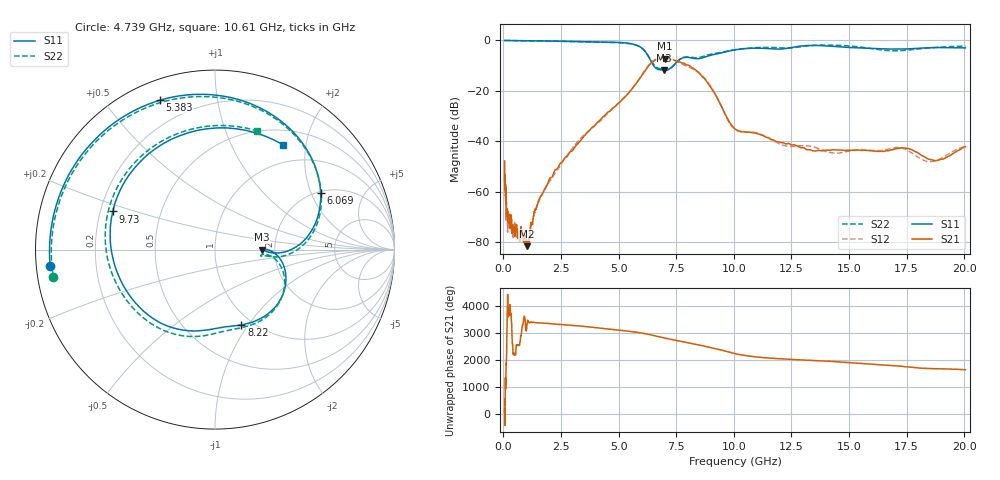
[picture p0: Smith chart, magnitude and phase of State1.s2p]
# Hz S DB R 50
!freq MagS11 AngS11 MagS21 AngS21 MagS12 AngS12 MagS22 AngS22
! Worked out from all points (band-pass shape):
!   1601 points, 50 MHz to 20.05 GHz, reference 50 ohm
!   highest |S21| = -7.19 dB at 7.024 GHz (marker M1); lowest = -81.5 dB at 1.016 GHz (marker M2)
!   |S21| within 3 dB of the highest: 6.292 GHz to 8.101 GHz (1.808 GHz wide, 25.1 % of centre)
!   lowest |S11| = -11.7 dB at 6.971 GHz (marker M3), VSWR 1.70, Z = 85.2 + j0.0103 ohm
!   |S11| at or under -10 dB: 6.519 GHz to 7.366 GHz (846.4 MHz wide, 12.2 % of centre)
!   |S22| runs from -11.8 to 0.0 dB; largest |S21 - S12| = 0.028
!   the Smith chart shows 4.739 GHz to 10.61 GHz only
!   S11 on the Smith chart (normalised r, x): 4.739 GHz: 0.04, -0.05; 5.383 GHz: 0.09, +0.69; 6.069 GHz: 2.06, +2.35; 8.22 GHz: 0.89, -0.93; 9.73 GHz: 0.25, +0.17; 10.61 GHz: 0.71, +1.61
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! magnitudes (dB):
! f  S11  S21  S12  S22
! 50 MHz  0.0  -47.8  -57.9  0.0
! 52.89 MHz  0.0  -55.3  -55.0  0.0
! 109 MHz  0.0  -61.2  -69.4  0.0
! 135.9 MHz  0.0  -68.4  -67.3  0.0
! 165.2 MHz  0.0  -68.3  -68.3  0.0
! 181.4 MHz  0.0  -68.6  -74.8  0.0
! 193.3 MHz  0.0  -69.3  -70.1  0.0
! 369.6 MHz  0.0  -75.1  -74.2  0.0
! 1.005 GHz  -0.1  -80.3  -79.9  -0.1
! 1.016 GHz  -0.1  -81.5  -81.0  -0.1
! 2.722 GHz  -0.3  -46.2  -46.1  -0.4
! 4.739 GHz  -0.7  -26.8  -27.0  -0.8
! 5.383 GHz  -1.0  -21.3  -21.3  -1.2
! 6.069 GHz  -3.5  -13.0  -12.8  -3.6
! 6.971 GHz  -11.7  -7.2  -7.0  -11.7
! 7.024 GHz  -11.7  -7.2  -7.0  -11.8
! 7.402 GHz  -9.7  -7.8  -7.9  -9.8
! 8.22 GHz  -7.0  -11.0  -11.3  -6.7
! 9.73 GHz  -4.3  -31.0  -31.3  -4.1
! 10.61 GHz  -3.1  -36.4  -36.3  -3.1
! 18.46 GHz  -2.9  -47.1  -48.0  -3.0
! 20.05 GHz  -2.9  -42.1  -42.1  -2.3
